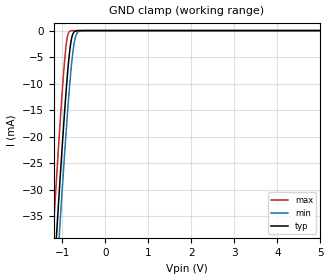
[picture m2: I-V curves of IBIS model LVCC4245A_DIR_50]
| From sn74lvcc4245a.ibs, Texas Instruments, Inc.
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[Model]   LVCC4245A_DIR_50
Model_type  Input
Vinl=0.8
Vinh=2.0
| variable   typ   min   max
C_comp   2.92pF   2.28pF   3.99pF
[Temperature Range]   40   100   -40
| Ambient temperature   25   85   -40
[Voltage range]   5   4.5   5.5
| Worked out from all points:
|   GND clamp passes 1 mA (typ) near -0.77 V on its own axis
[GND Clamp]
| LVCC4245A_DIR_50
|   Voltage   I(typ)   I(min)   I(max)
-5V       -584.4mA   -591.5mA   -575.7mA
-1.21V    -48.99mA   -57.28mA   -38.34mA
-1.13V    -38.46mA   -46.76mA   -27.8mA
-1.07V    -30.74mA   -39.01mA   -20.15mA
-1.05V    -28.22mA   -36.46mA   -17.67mA
-915mV    -12.22mA   -19.97mA   -3.336mA
-870mV    -7.659mA   -14.92mA   -892uA
-815mV    -3.256mA   -9.309mA   -87.15uA
-770mV    -1.129mA   -5.45mA    -10.74uA
-705mV    -146.9uA   -1.725mA   -505.6nA
-575mV    -1.598uA   -53.03uA   -1.119nA
5V        9.69pA     12.83pA    9.218pA
